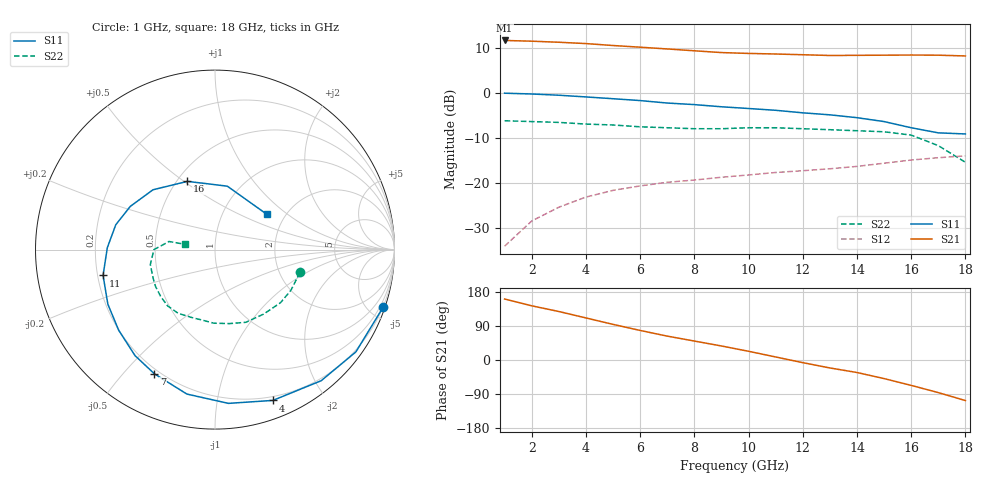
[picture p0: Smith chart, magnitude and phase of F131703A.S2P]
!ATF-13170
!S-PARAMETERS at Vds=2.5V  Id=20mA.  LAST UPDATED 07-22-92
# ghz s ma r 50
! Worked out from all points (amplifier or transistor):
!   18 points, 1 GHz to 18 GHz, reference 50 ohm
!   highest |S21| = 11.6 dB at 1 GHz (marker M1)
!   |S21| within 3 dB of that: start of sweep to 11 GHz
!   unconditionally stable (mu >= 1): 15.6 GHz to end of sweep
!   at 4 GHz: K = 0.39, MSG = 17.0 dB, |S12| = -23.1 dB
!   at 10 GHz: K = 0.81, MSG = 13.5 dB, |S12| = -18.2 dB
!   at 18 GHz: K = 1.07, MAG = 9.4 dB, |S12| = -14.0 dB
!   lowest NFmin = 0.50 dB at 4 GHz
!   S11 on the Smith chart (normalised r, x): 1 GHz: 0.18, -5.97; 4 GHz: 0.16, -1.44; 7 GHz: 0.18, -0.61; 11 GHz: 0.22, -0.11; 16 GHz: 0.56, +0.52; 18 GHz: 1.62, +0.72
1  0.99 -19.0  3.8 161.0  0.02 77.0  0.49 -15.0
2  0.97 -36.0  3.73 143.0  0.038 65.0  0.48 -28.0
3  0.94 -51.0  3.63 128.0  0.054 55.0  0.47 -39.0
4  0.9 -69.0  3.51 111.0  0.07 43.0  0.45 -53.0
5  0.86 -85.0  3.34 94.0  0.083 32.0  0.44 -67.0
6  0.82 -101.0  3.2 78.0  0.093 20.0  0.42 -79.0
7  0.77 -116.0  3.06 63.0  0.102 10.0  0.41 -91.0
8  0.74 -127.0  2.92 50.0  0.108 2.0  0.4 -99.0
9  0.7 -140.0  2.79 37.0  0.116 -7.0  0.4 -109.0
10  0.67 -153.0  2.73 23.0  0.123 -17.0  0.41 -120.0
11  0.64 -167.0  2.69 8.0  0.131 -28.0  0.41 -130.0
12  0.6 179.0  2.64 -7.0  0.137 -39.0  0.4 -139.0
13  0.57 166.0  2.59 -21.0  0.144 -50.0  0.39 -148.0
14  0.53 153.0  2.6 -33.0  0.153 -59.0  0.38 -155.0
15  0.48 136.0  2.61 -49.0  0.166 -73.0  0.37 -167.0
16  0.41 112.0  2.62 -67.0  0.18 -88.0  0.34 180.0
17  0.36 79.0  2.61 -86.0  0.191 -105.0  0.26 170.0
18  0.35 34.0  2.56 -107.0  0.2 -124.0  0.17 170.0
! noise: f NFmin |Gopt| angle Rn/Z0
4  0.5  0.62  56  0.44
6  0.7  0.47  81  0.34
8  0.8  0.53  116  0.19
12  1  0.44  157  0.12
14  1.3  0.43  179  0.07
